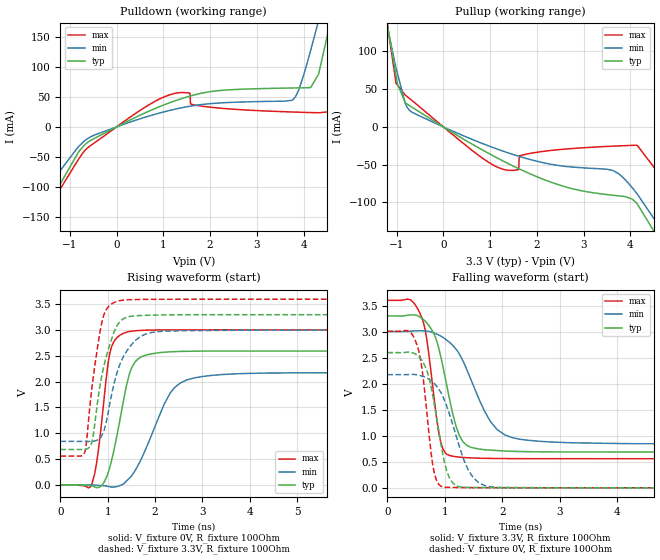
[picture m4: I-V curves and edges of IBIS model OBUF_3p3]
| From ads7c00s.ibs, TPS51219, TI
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|   Model
[Model]   OBUF_3p3
Model_type   Output
Polarity   Non-Inverting
Vmeas = 1.65
Vref = 0
Cref = 1pF
Rref = 10000
|   typ   min   max
C_comp   2.314pF   1.935pF   2.523pF
[Voltage Range]   3.3   3   3.6
[Temperature Range]   27   125   -40
[Pullup Reference]   3.3   3   3.6
[Pulldown Reference]   0   0   0
[Power Clamp Reference]   3.3   3   3.6
[GND Clamp Reference]   0   0   0
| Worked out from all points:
|   slope of the pulldown table from 0 to 0.495 V, typ, clamps not added: 25.6 ohm
|   slope of the pullup table from 0 to 0.495 V, typ, clamps not added: 26.8 ohm
|   falling waveform, V_fixture 3.3V, R_fixture 100Ohm: 20-80 % time 318ps typ, 541ps min, 216ps max; typ from 3.3 V to 0.686 V
|   rising waveform, V_fixture 0V, R_fixture 100Ohm: 20-80 % time 345ps typ, 624ps min, 223ps max; typ from 0 V to 2.6 V
|   rising waveform, V_fixture 3.3V, R_fixture 100Ohm: 20-80 % time 334ps typ, 402ps min, 256ps max; typ from 0.686 V to 3.3 V
|   falling waveform, V_fixture 0V, R_fixture 100Ohm: 20-80 % time 255ps typ, 400ps min, 183ps max; typ from 2.6 V to 0 V
[Pulldown]
|   Voltage   I(typ)   I(min)   I(max)
-3.3V     -1.547A    -1.4A      -1.656A
-1.924V   -249.9mA   -167.1mA   -325.9mA
-1.726V   -166.7mA   -127.6mA   -179.7mA
-676.5mV  -29.61mA   -22.8mA    -39.29mA
1.125V    40.16mA    27.38mA    53.54mA
3.769V    65.16mA    45.26mA    24.96mA
4.155V    65.93mA    128.4mA    24.04mA
4.323V    88.25mA    178mA      23.67mA
4.551V    167.2mA    247.9mA    25.32mA
4.67V     212.7mA    285.7mA    59.72mA
4.867V    290.8mA    350.8mA    156.4mA
6.6V      1.024A     945.9mA    1.104A
[Pullup]
|   Voltage   I(typ)   I(min)   I(max)
-3.3V     1.024A     841.9mA    1.283A
-1.191V   131.9mA    130.4mA    133mA
-1.013V   67.51mA    77.65mA    57.75mA
-726mV    28.19mA    21.98mA    37.72mA
1.125V    -40.25mA   -28.71mA   -52.4mA
1.61V     -55.25mA   -38.77mA   -56.41mA
1.878V    -62.72mA   -43.48mA   -34.74mA
3.62V     -90.38mA   -57.5mA    -25.48mA
4.145V    -101.6mA   -88.62mA   -24.26mA
4.709V    -158.7mA   -140.1mA   -69.81mA
5.214V    -253.9mA   -375.6mA   -140.7mA
6.6V      -1.548A    -1.693A    -1.36A
[Ramp]
R_load = 100
|   typ   min   max
dV/dt_r   1.55762/3.44526e-10   1.30401/6.23651e-10   1.80351/2.23398e-10
dV/dt_f   1.56856/3.17578e-10   1.29475/5.41349e-10   1.82553/2.15851e-10
[Falling Waveform]
V_fixture = 3.3V
V_fixture_min = 3V
V_fixture_max = 3.6V
R_fixture = 100Ohm
C_fixture = 0F
|   Time   V(typ)   V(min)   V(max)
0s        3.3V       3V         3.6V
397.3ps   3.317V     3.006V     3.613V
582.2ps   3.268V     3.016V     3.316V
689.2ps   3.162V     3.009V     2.83V
926.4ps   2.536V     2.916V     891.3mV
1.116ns   1.532V     2.759V     611.2mV
1.39ns    810.1mV    2.252V     579.4mV
1.909ns   716.5mV    1.12V      563.3mV
2.417ns   695.5mV    917.8mV    560mV
15ns      685.7mV    842.1mV    557.5mV
[Rising Waveform]
V_fixture = 0V
V_fixture_min = 0V
V_fixture_max = 0V
R_fixture = 100Ohm
C_fixture = 0F
|   Time   V(typ)   V(min)   V(max)
0s        311.1nV    238.3nV    23.45nV
666.5ps   -22.74mV   -2.934mV   22.82mV
790.6ps   -53mV      -10.08mV   593.6mV
1.043ns   342.4mV    -38.01mV   2.551V
1.159ns   794.4mV    -39.28mV   2.816V
1.424ns   2.027V     97.93mV    2.966V
1.645ns   2.445V     389mV      2.991V
2.318ns   2.579V     1.777V     3.003V
2.974ns   2.593V     2.097V     3.004V
15ns      2.596V     2.173V     3.006V
[Rising Waveform]
V_fixture = 3.3V
V_fixture_min = 3V
V_fixture_max = 3.6V
R_fixture = 100Ohm
C_fixture = 0F
|   Time   V(typ)   V(min)   V(max)
0s        685.7mV    842.1mV    557.2mV
515.9ps   686.1mV    840.3mV    635.3mV
552.6ps   694.2mV    839.9mV    837.7mV
660.6ps   812.2mV    842.7mV    1.846V
893.2ps   2.2V       995.5mV    3.222V
1.134ns   2.967V     1.966V     3.534V
1.259ns   3.165V     2.339V     3.573V
1.69ns    3.282V     2.873V     3.593V
2.188ns   3.293V     2.978V     3.597V
15ns      3.3V       3V         3.6V
[Falling Waveform]
|Gnd
V_fixture = 0V
V_fixture_min = 0V
V_fixture_max = 0V
R_fixture = 100Ohm
C_fixture = 0F
|   Time   V(typ)   V(min)   V(max)
0s        2.596V     2.173V     3.006V
378.6ps   2.604V     2.176V     3.005V
515.9ps   2.551V     2.168V     2.744V
606ps     2.437V     2.145V     2.262V
790.6ps   1.777V     2.03V      437mV
963.6ps   656.6mV    1.758V     18.13mV
1.134ns   98.53mV    1.23V      8.393mV
1.408ns   8.142mV    343mV      4.881mV
1.795ns   4.591mV    19.46mV    2.706mV
15ns      157.2nV    -3.624uV   220.7nV
